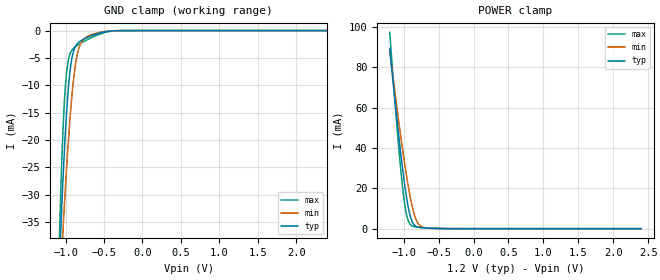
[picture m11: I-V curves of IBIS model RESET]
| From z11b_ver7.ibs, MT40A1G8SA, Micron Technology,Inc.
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| MODEL RESET (RESET_n Input Model)
[Model]   RESET
Model_type   Input
Vinl = 240.000mV
Vinh = 960.000mV
|   typ   min   max
|C_comp   0.300pF   0.250pF   0.350pF
C_comp_power_clamp   0.1500pF   0.1250pF   0.1750pF
C_comp_gnd_clamp   0.1500pF   0.1250pF   0.1750pF
[Model Spec]
| Input threshold voltage corners
Vinl   0.2400V   0.2280V   0.2520V
Vinh   0.9600V   0.9120V   1.0080V
[Voltage Range]   1.2000V   1.1400V   1.2600V
| Junction Temperature (Ambient temp is 35C typ, 95C min, 0C max)
[Temperature Range]   50.0   110.0   0.0
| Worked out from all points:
|   GND clamp passes 1 mA (typ) near -0.67 V on its own axis
|   POWER clamp passes 1 mA (typ) near -0.81 V on its own axis
[GND Clamp]
|   Voltage   I(typ)   I(min)   I(max)
-1.2V     -89.68mA   -83.76mA   -112.5mA
-1.08V    -42.27mA   -48.6mA    -37.43mA
-1.065V   -37.02mA   -44.48mA   -30.24mA
-1.035V   -27.36mA   -36.67mA   -18.41mA
-1.015V   -21.61mA   -31.62mA   -12.71mA
-990mV    -15.4mA    -25.73mA   -8.028mA
-935mV    -6.48mA    -14.64mA   -4.005mA
-875mV    -2.985mA   -6.456mA   -2.943mA
-820mV    -2.025mA   -2.921mA   -2.441mA
-715mV    -1.243mA   -1.044mA   -1.636mA
-425mV    -95.71uA   -64.44uA   -150uA
2.4V      0A         0A         0A
[POWER Clamp]
|   Voltage   I(typ)   I(min)   I(max)
-1.2V     89.29mA    88mA       97.25mA
-1.095V   53.78mA    59.42mA    50.04mA
-1.05V    39.66mA    47.81mA    32.16mA
-1.015V   29.47mA    39.09mA    20.17mA
-985mV    21.54mA    31.96mA    11.96mA
-955mV    14.57mA    25.34mA    6.252mA
-925mV    9.043mA    19.2mA     3.084mA
-890mV    4.569mA    12.96mA    1.546mA
-850mV    1.945mA    7.193mA    981.4uA
-805mV    853.4uA    3.217mA    763.2uA
-665mV    277.9uA    269.6uA    403.6uA
2.4V      0A         0A         0A
